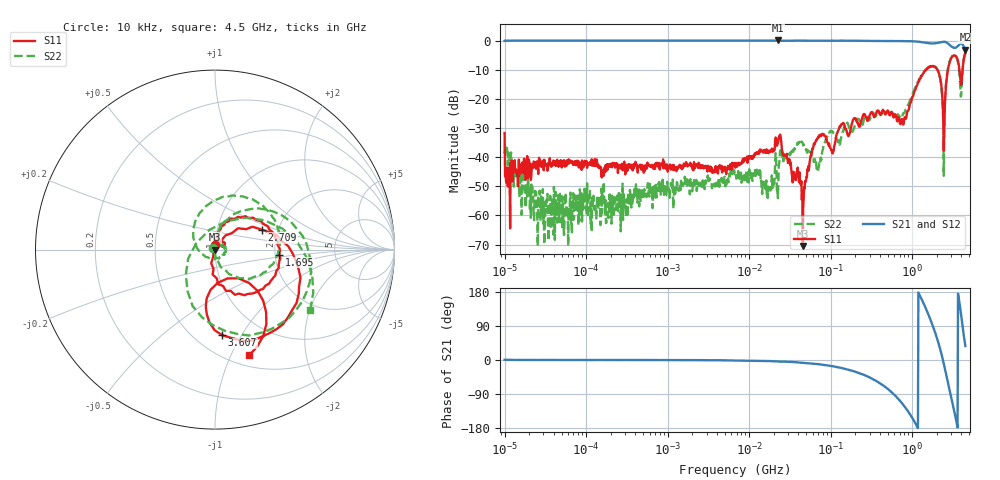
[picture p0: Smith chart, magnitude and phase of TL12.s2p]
!Siglent Technologies,SNA5004A,SNA5XCED5R0097,V1.0.0.2.10.R9
!Date: 2024-11-24 17:30:07
!Data & Calibration Information:
!Freq	S11:F2(ON)	S21:F2(ON)	S12:F2(ON)	S22:F2(ON)
# Hz S DB R 50
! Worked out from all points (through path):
!   1001 points, 10 kHz to 4.5 GHz, reference 50 ohm
!   highest |S21| = 0.10 dB at 22.8 MHz (marker M1); lowest = -3.1 dB at 4.5 GHz (marker M2)
!   group delay of S21, straight-line fit = 420 ps
!   lowest |S11| = -70.5 dB at 45.46 MHz (marker M3), VSWR 1.00, Z = 50 + j0.0279 ohm
!   |S11| at or under -10 dB: start of sweep to 1.473 GHz; 2.044 GHz to 2.75 GHz (705.8 MHz wide, 29.4 % of centre); 3.805 GHz to 4.15 GHz (345.4 MHz wide, 8.68 % of centre)
!   |S22| runs from -70.6 to -4.0 dB; largest |S21 - S12| = 0.023
!   S11 on the Smith chart (normalised r, x): 10 kHz: 1.00, +0.05; 1.695 GHz: 2.11, -0.13; 2.709 GHz: 1.65, +0.40; 3.607 GHz: 0.67, -0.83; 4.5 GHz: 0.62, -1.18
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10000  -31.68 84.9  -0.02 0.8  -0.04 0.8  -38.73 137.4
10953.99  -50.10 28.9  0.04 0.3  -0.01 0.2  -42.78 82.9
23920.22  -41.90 5.0  0.06 0.1  0.01 -0.0  -53.78 118.2
87919.76  -44.35 8.5  0.05 0.0  0.00 -0.1  -51.85 -71.4
772988.4  -43.39 15.5  0.06 -0.1  0.01 -0.3  -48.89 -54.5
6708204  -42.81 64.5  0.04 -1.0  -0.03 -1.2  -45.88 -134.5
1.757697e7  -37.72 108.3  0.04 -2.8  -0.04 -2.8  -50.55 -41.1
2.280385e7  -34.62 124.0  0.10 -3.8  0.03 -3.7  -49.37 139.9
4.54599e7  -70.52 110.3  0.05 -7.1  -0.05 -7.1  -35.08 87.2
5.897837e7  -38.38 44.0  0.01 -9.3  -0.06 -9.3  -39.01 116.7
2.343869e8  -28.10 53.2  -0.03 -35.9  -0.10 -35.7  -28.37 51.7
5.185364e8  -25.06 34.8  -0.09 -78.8  -0.15 -78.6  -24.88 -12.7
7.563493e8  -27.08 50.1  -0.12 -114.9  -0.16 -114.6  -25.97 -107.2
1.117683e9  -15.92 69.4  -0.26 -170.5  -0.30 -170.2  -15.42 134.5
1.695202e9  -8.90 -4.5  -0.90 103.7  -0.96 104.2  -8.65 33.5
2.286891e9  -15.83 -86.3  -0.45 16.3  -0.51 16.8  -15.97 -59.9
2.505059e9  -24.75 56.5  -0.36 -20.0  -0.42 -19.4  -22.85 88.3
2.708552e9  -10.91 22.9  -0.80 -54.0  -0.86 -53.4  -10.73 50.2
3.125522e9  -5.30 -33.2  -2.22 -115.0  -2.26 -114.1  -5.20 -13.4
3.606682e9  -6.40 -85.2  -1.95 -178.2  -2.01 -177.2  -6.80 -82.8
4.054962e9  -13.69 -50.8  -0.98 106.9  -1.02 108.1  -15.36 68.0
4.5e9  -4.16 -72.0  -3.06 36.7  -3.11 38.0  -4.03 -32.5
